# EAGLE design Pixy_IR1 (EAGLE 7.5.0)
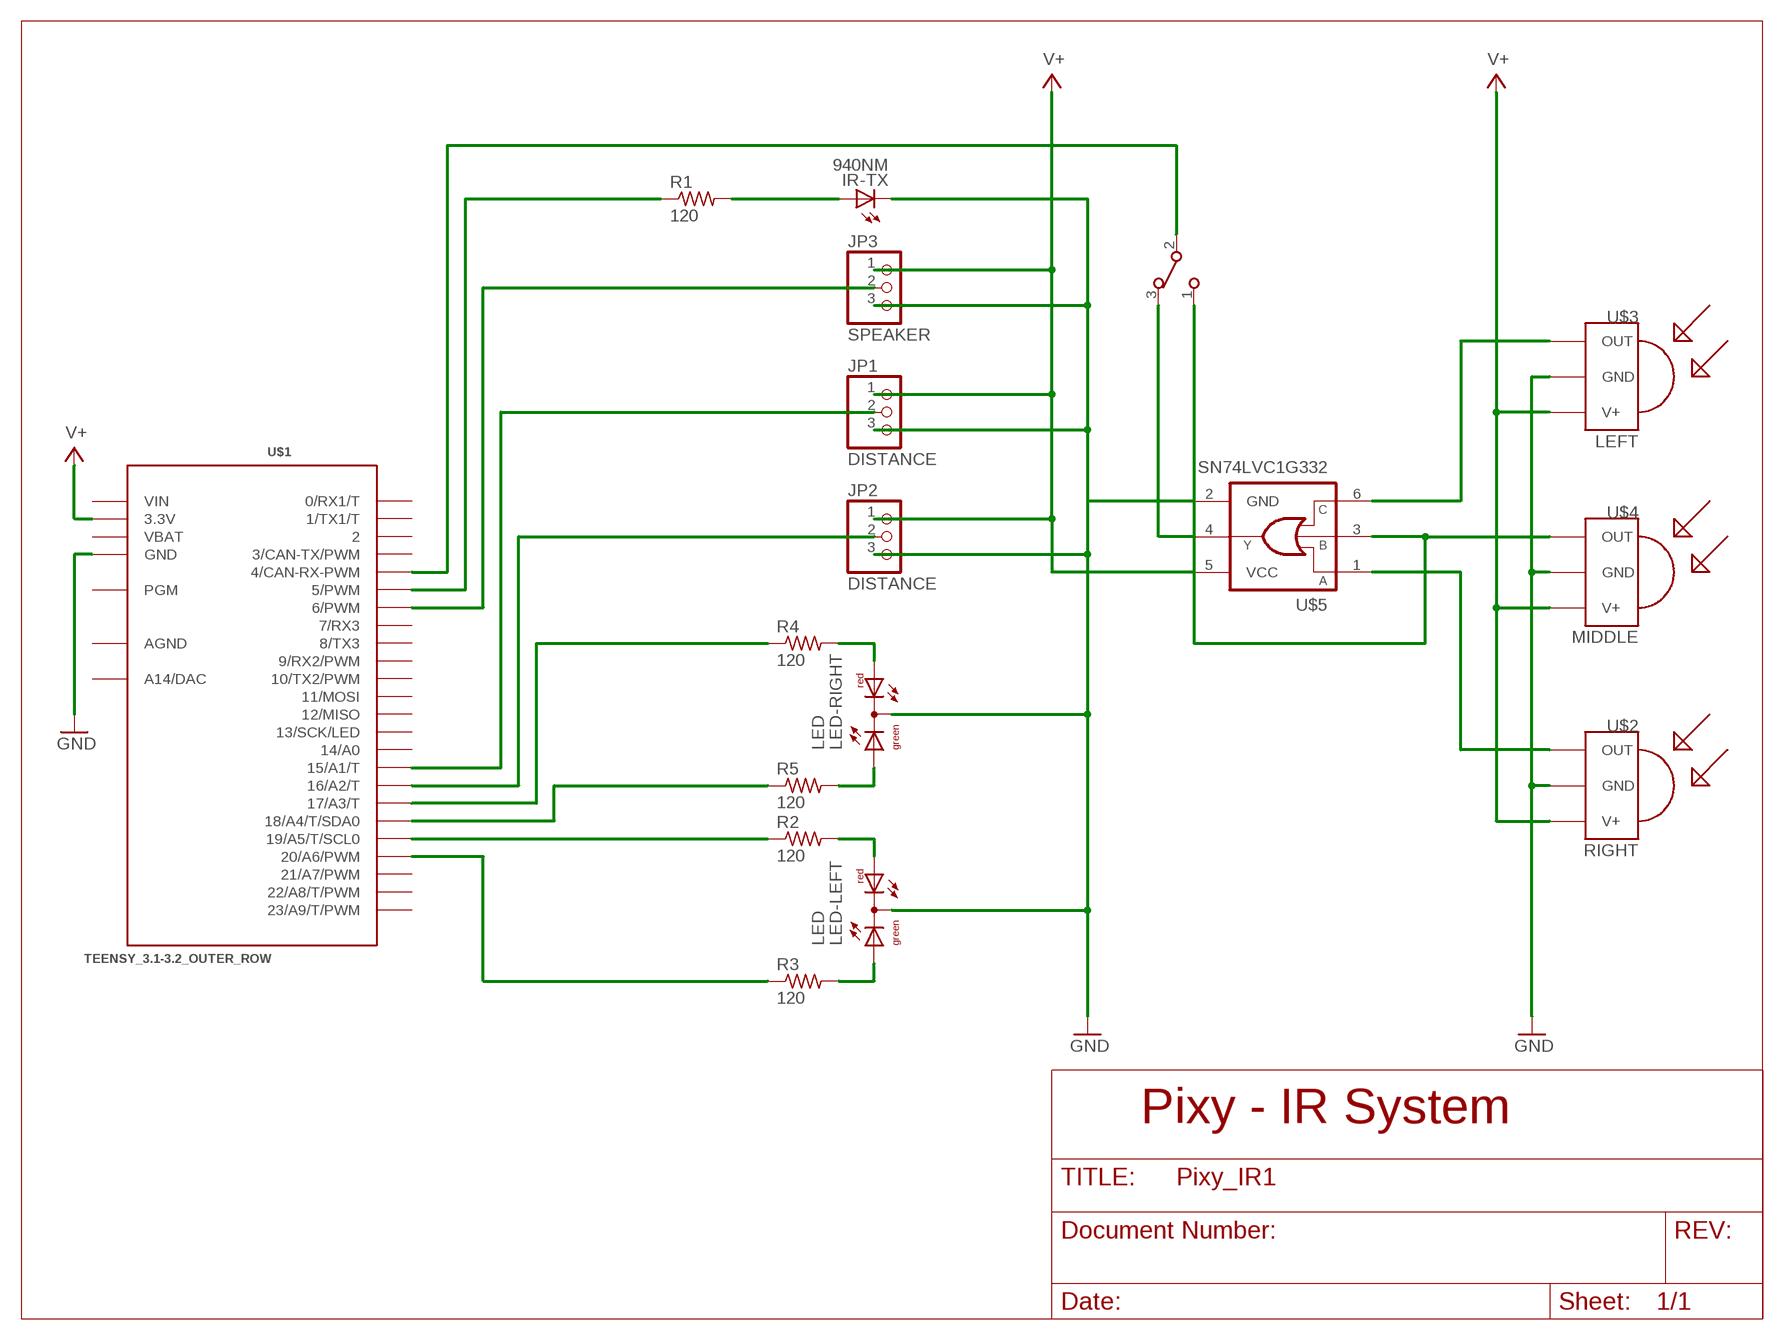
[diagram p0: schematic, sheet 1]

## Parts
IR-TX  940NM  LED5MM  [LED5MM]
JP1  DISTANCE  PINHD-1X3  [1X03]
JP2  DISTANCE  PINHD-1X3  [1X03]
JP3  SPEAKER  PINHD-1X3  [1X03]
LED-LEFT  LED  DUOLED-RG-C  [DUOLED-C-5MM]
LED-RIGHT  LED  DUOLED-RG-C  [DUOLED-C-5MM]
R1  120  R-US_R1206  [R1206]
R2  120  R-US_R1206  [R1206]
R3  120  R-US_R1206  [R1206]
R4  120  R-US_R1206  [R1206]
R5  120  R-US_R1206  [R1206]
SW1  CAS-120CAS-120B1  [CAS-120B1]
U$1  TEENSY_3.1-3.2_OUTER_ROW  [TEENSY_3.0-3.2&LC_OUTER_ROW]
U$2  RIGHT  TSOP3X  [TSOP18XX]
U$3  LEFT  TSOP3X  [TSOP18XX]
U$4  MIDDLE  TSOP3X  [TSOP18XX]
U$5  SN74LVC1G332  [SC70-6]

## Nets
GND: IR-TX.K(C) JP1.3 JP2.3 JP3.3 LED-LEFT.C LED-RIGHT.C U$1.GND U$1.GND1(GND) U$2.GND U$3.GND U$4.GND U$5.2(GND)
N$1: R2.1 U$1.19/A5(19/A5/T/SCL0)
N$2: R5.1 U$1.18/A4(18/A4/T/SDA0)
N$3: LED-RIGHT.AR R4.2
N$4: LED-RIGHT.AX(AG) R5.2
N$5: LED-LEFT.AR R2.2
N$6: LED-LEFT.AX(AG) R3.2
N$7: JP3.2 U$1.6(6/PWM)
N$8: R1.1 U$1.5(5/PWM)
N$9: R4.1 U$1.17/A3(17/A3/T)
N$10: R3.1 U$1.20/A6(20/A6/PWM)
N$11: JP1.2 U$1.15/A1(15/A1/T)
N$12: IR-TX.A R1.2
N$13: JP2.2 U$1.16/A2(16/A2/T)
N$14: SW1.2 U$1.4(4/CAN-RX-PWM)
N$15: SW1.3 U$5.4(Y)
N$16: SW1.1 U$4.OUT U$5.3(B)
N$17: U$3.OUT U$5.6(C)
N$18: U$2.OUT U$5.1(A)
V+: JP1.1 JP2.1 JP3.1 U$1.3.3V U$1.3.3V1(3.3V) U$2.VCC(V+) U$3.VCC(V+) U$4.VCC(V+) U$5.5(VCC)
Unconnected: U$1.0(0/RX1/T) U$1.1(1/TX1/T) U$1.2 U$1.3(3/CAN-TX/PWM) U$1.7(7/RX3) U$1.8(8/TX3) U$1.9(9/RX2/PWM) U$1.10(10/TX2/PWM) U$1.11(11/MOSI) U$1.12(12/MISO) U$1.13(13/SCK/LED) U$1.14/A0 U$1.21/A7(21/A7/PWM) U$1.22/A8(22/A8/T/PWM) U$1.23/A9(23/A9/T/PWM) U$1.PGM U$1.RESET/DAC(A14/DAC)

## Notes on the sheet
- Pixy - IR System

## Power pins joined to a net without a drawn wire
AGND: U$1.AGND
VBAT: U$1.VBAT
VIN: U$1.VIN

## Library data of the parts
IR-TX = led:LED: LED
JP1-JP3 = pinhead:PINHD-1X3: PIN HEADER
LED-LEFT LED-RIGHT = led:DUOLED-RG-C: DUO LED 2 colors (red/green), 5 mm, round, common Cathode www.ligitek.com or other producers.
R1-R5 = resistor:R-US_: RESISTOR, American symbol
SW1 = Switch2:CAS-120: CAS-120 surface mount type slide switch Producted by COPAL ELECTRONICS Store Information : Digi-Key : http://search.digikey.com/scripts/DkSearch/dksus.dll?Detail&name=CAS120GCT-ND
U$1 = Teensy_3_and_LC_Series_Boards_v1.4:TEENSY_3.1-3.2_OUTER_ROW: Footprint for Teensy 3.1 or 3.2 board using all pin connections on the outer perimeter
U$2-U$4 = _Loper:TSOP3X: IR Receiver and Demodulator
U$5 = 74LV:SN74LVC1G332: OR GATE 3-INPUT

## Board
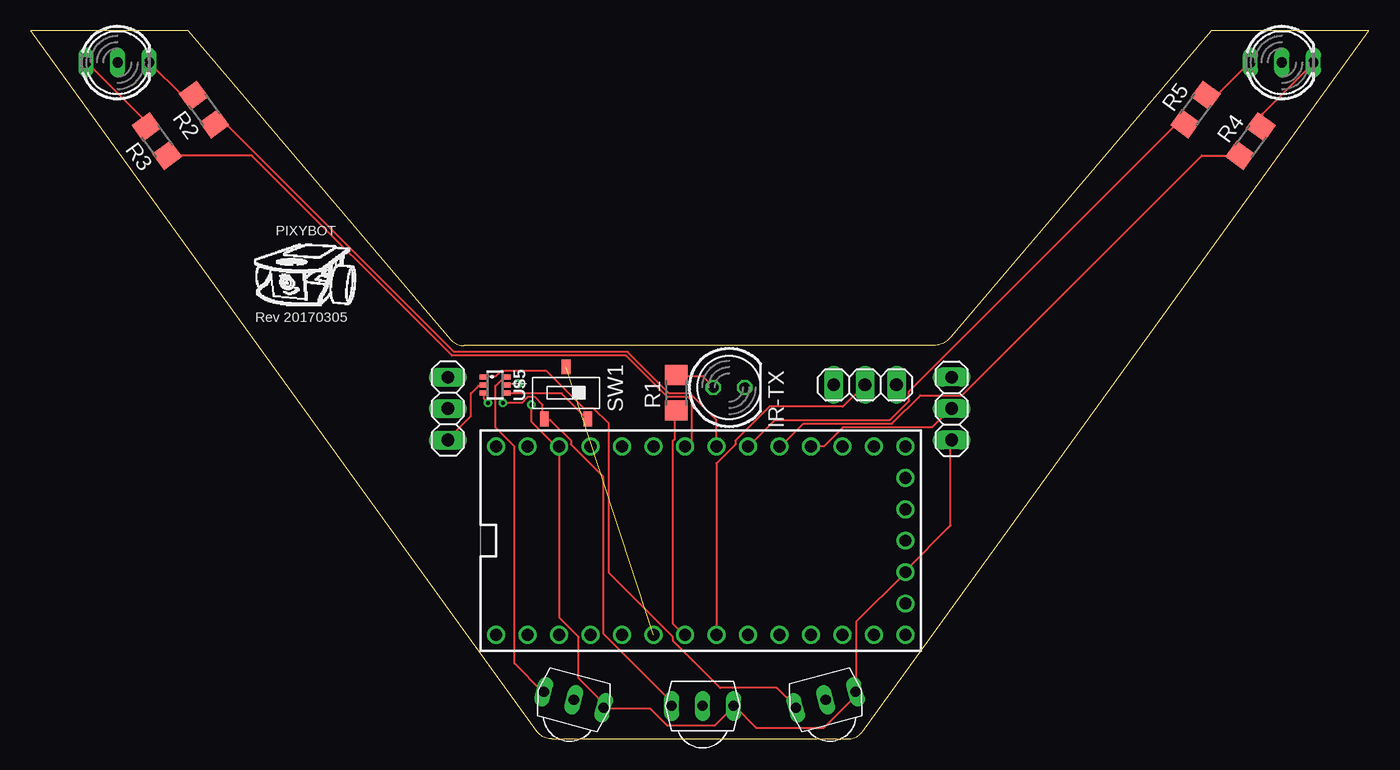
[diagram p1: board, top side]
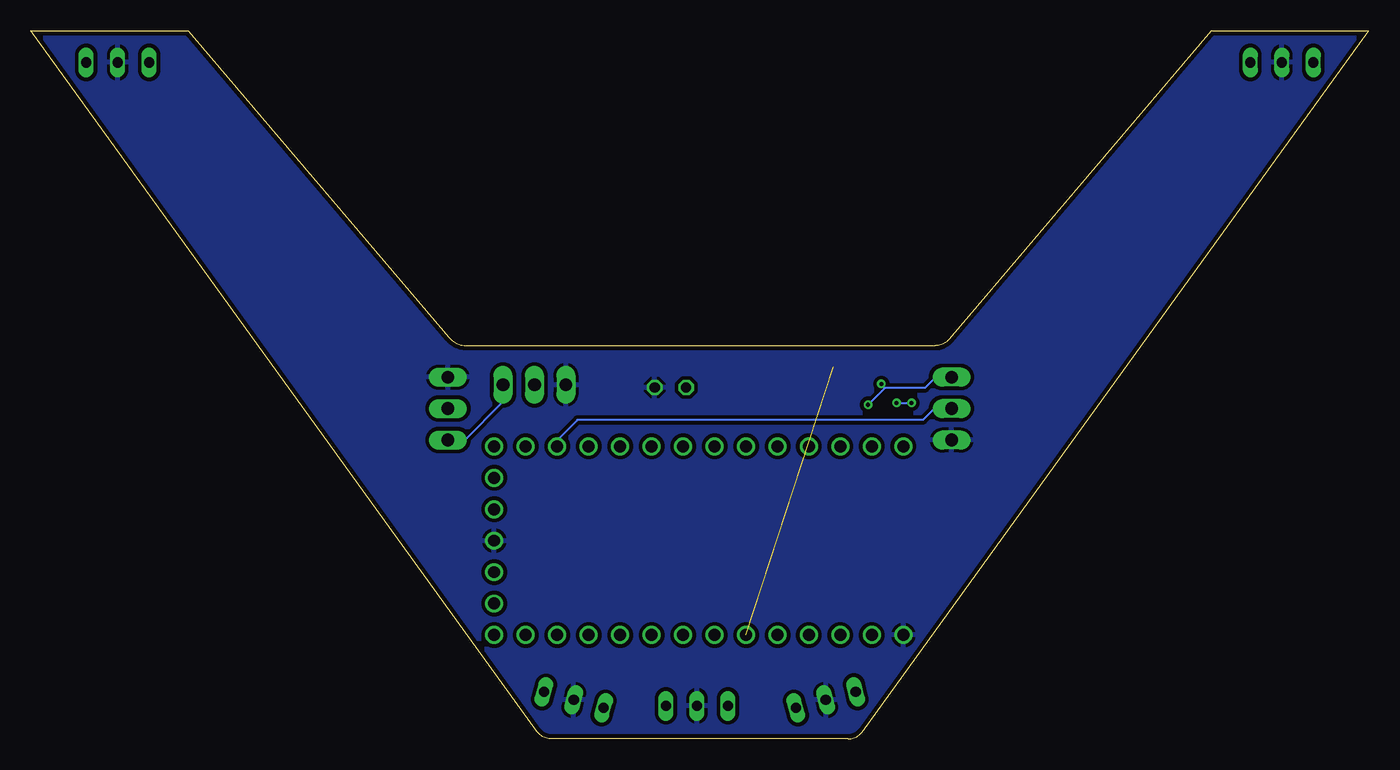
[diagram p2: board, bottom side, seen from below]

Size 107.95 x 57.15 mm. Coordinates in mm from the lower left corner, seen from the top.
Outline: 42,0 65.95,0 arc54 67.1,0.59 107.95,57.15 95.25,57.15 74.2,32.38 arc-50 72.83,31.75 34.95,31.75 arc-50 33.87,32.25 12.7,57.15 0,57.15 40.85,0.59 arc54 42,0
Copper layers (1*16): Top 0.0356mm / dielectric 1.5011mm / Bottom 0.0356mm
Design rules "oshpark-2layer": minimum track width 6mil, minimum drill 13mil, track to track 6mil, track to pad 6mil, pad to pad 6mil, via to via 6mil, smd to smd 6mil, copper to edge 15mil, drill to drill 6mil, minimum pad ring 7mil, minimum via ring 7mil, stop-mask expansion 2.5mil, vias tented up to drill 0mil, thermal gap 10mil

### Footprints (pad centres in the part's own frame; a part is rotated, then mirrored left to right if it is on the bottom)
LED5MM = drill 0.813 octagon: A -1.27,0; K 1.27,0
1X03 = drill 1.016 long: 1 -2.54,0; 2 0,0; 3 2.54,0
DUOLED-C-5MM = drill 0.813 long: AR 2.54,0; AX -2.54,0; C 0,0
R1206 = smd 1.6 x 1.803: 1 -1.422,0; 2 1.422,0
CAS-120B1 = smd 0.7 x 1.2: 1 -1.75,-2.1; 2 0,2.1; 3 1.75,-2.1
TEENSY_3.0-3.2&LC_OUTER_ROW = drill 0.965: 0 -7.62,13.97; 1 -7.62,11.43; 2 -7.62,8.89; 3 -7.62,6.35; 3.3V 7.62,11.43; 3.3V1 -2.54,-16.51; 4 -7.62,3.81; 5 -7.62,1.27; 6 -7.62,-1.27; 7 -7.62,-3.81; 8 -7.62,-6.35; 9 -7.62,-8.89; 10 -7.62,-11.43; 11 -7.62,-13.97; 12 -7.62,-16.51; 13 7.62,-16.51; 14/A0 7.62,-13.97; 15/A1 7.62,-11.43; 16/A2 7.62,-8.89; 17/A3 7.62,-6.35; 18/A4 7.62,-3.81; 19/A5 7.62,-1.27; 20/A6 7.62,1.27; 21/A7 7.62,3.81; 22/A8 7.62,6.35; 23/A9 7.62,8.89; AGND 7.62,13.97; GND -7.62,16.51; GND1 0,-16.51; PGM 2.54,-16.51; RESET/DAC 5.08,-16.51; VBAT -5.08,-16.51; VIN 7.62,16.51
TSOP18XX = drill 0.813 long: GND -0.001,-0.027; OUT -2.501,-0.027; VCC 2.499,-0.027
SC70-6 = smd 0.4 x 0.6: 1 -0.65,-0.95; 2 0,-0.95; 3 0.65,-0.95; 4 0.65,0.95; 5 0,0.95; 6 -0.65,0.95

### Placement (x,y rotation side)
IR-TX  56.34,28.37 0 top
JP1  33.66,26.67 270 top
JP2  74.3,26.67 90 top
JP3  67.31,28.57 180 top
LED-LEFT  6.99,54.61 0 top
LED-RIGHT  100.97,54.61 0 top
R1  52.07,27.94 90 top
R2  13.97,50.8 126 top
R3  10.16,48.26 126 top
R4  98.42,48.26 54 top
R5  93.98,50.8 54 top
SW1  43.18,27.94 0 top
U$1  54.05,16 90 top
U$2  64.14,3.17 15 top
U$3  43.81,3.17 345 top
U$4  54.2,2.69 0 top
U$5  37.47,28.57 270 top

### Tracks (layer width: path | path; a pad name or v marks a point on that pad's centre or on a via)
GND
  Top 0.152: U$5.2 36.42,28.5 36.12,28.5 35.51,27.89 35.51,26.06 33.68,24.23 JP1.3
  pour Bottom (isolate 0.305): 0,57.15 12.7,57.15 34.29,31.75 73.66,31.75 95.25,57.15 107.95,57.15 66.67,0 41.27,0
N$1
  Top 0.152: U$1.19/A5 55.32,25.76 53.19,27.89 51.51,27.89 48.16,31.24 34.14,31.24 15.85,49.53 14.94,49.53 R2.1
N$2
  Top 0.152: R5.1 93.12,49.53 92.35,49.53 70.87,28.04 70.87,27.28 69.34,25.76 60.05,25.76 57.91,23.62 U$1.18/A4
N$3
  Top 0.152: R4.2 99.36,49.53 99.36,50.44 103.48,54.56 LED-RIGHT.AR
N$4
  Top 0.152: R5.2 94.94,51.97 95.71,51.97 98.3,54.56 LED-RIGHT.AX
N$5
  Top 0.152: R2.2 13.11,51.97 12.19,51.97 9.6,54.56 LED-LEFT.AR
N$6
  Top 0.152: R3.2 9.3,49.53 9.3,49.84 4.57,54.56 LED-LEFT.AX
N$7
  Top 0.152: U$1.6 55.32,22.25 56.84,23.77 56.84,24.08 59.59,26.82 65.53,26.82 67.21,28.5 JP3.2
N$8
  Top 0.152: R1.1 51.97,26.52 51.97,24.23 51.82,24.08 51.82,9.3 52.73,8.38 U$1.5
N$9
  Top 0.152: R4.1 97.54,47.09 94.49,47.09 75.13,27.74 71.78,27.74 69.49,25.45 62.33,25.45 60.5,23.62 U$1.17/A3
N$10
  Top 0.152: R3.1 11.12,47.09 17.83,47.09 33.98,30.94 48.01,30.94 51.36,27.58 53.03,27.58 53.34,27.28 53.34,24.08 52.88,23.62 U$1.20/A6
N$11
  Bottom 0.152: JP1.2 35.05,26.67 35.97,25.76 63.86,25.76 65.38,24.23 65.38,23.62 U$1.15/A1
N$12
  Top 0.152: R1.2 52.12,29.26 54.25,29.26 55.02,28.5 IR-TX.A
N$13
  Top 0.152: U$1.16/A2 64.01,23.62 65.53,25.15 72.69,25.15 74.22,26.67 JP2.2
N$14  (1 unrouted)
N$15
  Top 0.152: U$5.4 38.56,27.89 42.82,27.89 44.81,25.91 SW1.3
N$16  (via drill 0.33)
  Top 0.152: v36.88,27.13 36.58,27.43 36.58,27.89 U$5.3 | v38.1,27.13 39.62,27.13 40.08,27.58 40.69,27.58 41.3,26.98 41.3,25.91 SW1.1 41.45,25.76 41.91,25.76 43.59,24.08 43.59,23.77 46.18,21.18 46.18,8.53 51.66,3.05 51.66,2.74 U$4.OUT
  Bottom 0.152: v38.1,27.13 v36.88,27.13
N$17
  Top 0.152: U$5.6 38.41,29.11 38.1,29.11 37.49,28.5 37.49,25.15 39.01,23.62 39.01,6.1 41.3,3.81 U$3.OUT
N$18
  Top 0.152: U$5.1 36.58,29.26 37.49,29.26 37.95,29.72 41.6,29.72 44.65,26.67 45.41,26.67 46.63,25.45 46.63,13.41 51.82,8.23 51.82,7.92 55.63,4.12 60.2,4.12 61.72,2.59 U$2.OUT
V+  (via drill 0.33)
  Top 0.152: JP2.1 74.22,24.08 74.22,17.22 70.56,13.56 U$1.3.3V1 70.56,13.41 66.6,9.45 66.6,3.81 U$2.VCC 66.45,3.66 66.45,3.35 64.01,0.91 58.52,0.91 56.84,2.59 U$4.VCC 56.69,2.59 55.17,1.07 51.36,1.07 49.99,2.44 46.33,2.44 U$3.VCC 46.18,2.59 46.18,2.9 44.2,4.88 44.2,8.23 42.67,9.75 42.67,23.62 U$1.3.3V 42.37,23.62 40.39,25.6 v40.39,26.98 | v39.32,28.65 38.56,28.65 U$5.5
  Bottom 0.152: JP3.1 69.95,28.5 69.95,27.13 72.85,24.23 74.22,24.23 JP2.1 | 39.01,28.35 v39.32,28.65 | 39.01,28.35 35.81,28.35 35.05,29.11 33.68,29.11 JP1.1 | v40.39,26.98 39.01,28.35

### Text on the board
tPlace: PIXYBOT | Rev 20170305

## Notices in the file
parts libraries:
74LV: Copyright (C) 2008, Bob Starr
